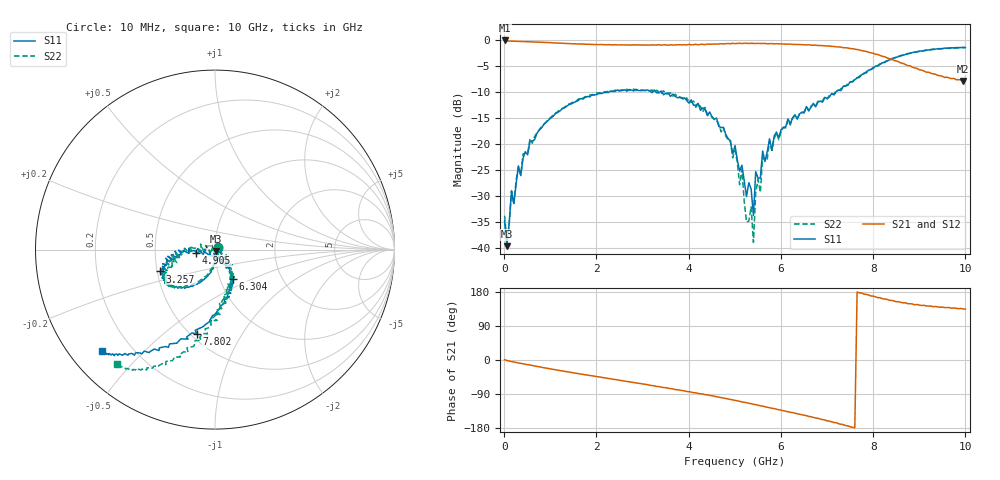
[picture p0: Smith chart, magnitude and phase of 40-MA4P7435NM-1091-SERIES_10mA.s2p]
!Agilent Technologies,E8364C,MY48140145,A.09.42.15
!Agilent E8364C: A.09.42.15
!Date: Wednesday, December 02, 2020 13:40:49
!Correction: S11(Full 2 Port(1,2))
!S21(Full 2 Port(1,2))
!S12(Full 2 Port(1,2))
!S22(Full 2 Port(1,2))
!S2P File: Measurements: S11, S21, S12, S22:
# Hz S  dB  R 50
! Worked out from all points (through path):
!   201 points, 10 MHz to 10 GHz, reference 50 ohm
!   highest |S21| = -0.11 dB at 10 MHz (marker M1); lowest = -7.9 dB at 9.95 GHz (marker M2)
!   group delay of S21, straight-line fit = 66.1 ps
!   lowest |S11| = -39.6 dB at 59.95 MHz (marker M3), VSWR 1.02, Z = 50.6 - j0.834 ohm
!   |S11| at or under -10 dB: start of sweep to 2.191 GHz; 3.293 GHz to 3.38 GHz (87.41 MHz wide, 2.62 % of centre); 3.42 GHz to 7.193 GHz (3.774 GHz wide, 71.1 % of centre)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
!   |S22| runs from -38.9 to -1.5 dB; largest |S21 - S12| = 0.021
!   S11 on the Smith chart (normalised r, x): 10 MHz: 1.03, +0.01; 3.257 GHz: 0.52, -0.14; 4.905 GHz: 0.81, -0.03; 6.304 GHz: 1.15, -0.39; 7.802 GHz: 0.54, -0.65; 10 GHz: 0.10, -0.38
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1e7  -34.80 20.2  -0.11 0.9  -0.16 -0.2  -33.77 44.9
5.995e7  -39.61 -51.9  -0.21 -1.5  -0.21 -1.6  -38.55 -59.8
1.5985e8  -29.03 -76.8  -0.24 -4.2  -0.24 -4.2  -28.99 -74.5
5.5945e8  -19.49 -97.6  -0.38 -13.6  -0.38 -13.6  -19.00 -97.4
1.7083e9  -11.37 -129.0  -0.80 -38.0  -0.78 -37.8  -11.18 -132.1
3.25675e9  -9.62 -158.4  -0.99 -68.2  -0.96 -68.9  -10.12 -150.0
3.35665e9  -10.17 -159.8  -0.94 -70.3  -0.96 -70.7  -9.99 -150.4
4.9051e9  -19.52 -169.8  -0.74 -104.3  -0.72 -103.8  -19.30 173.2
5.005e9  -20.30 177.0  -0.72 -106.6  -0.67 -106.6  -21.23 158.7
5.15485e9  -24.06 -171.5  -0.70 -110.6  -0.66 -110.5  -24.86 156.6
5.25475e9  -30.08 -167.5  -0.65 -112.8  -0.62 -113.0  -34.99 133.7
5.35465e9  -28.63 -88.2  -0.65 -115.2  -0.66 -115.3  -32.07 -59.1
5.4046e9  -33.69 -105.3  -0.67 -116.8  -0.65 -117.0  -38.88 29.5
5.45455e9  -25.30 -80.0  -0.69 -117.9  -0.69 -117.8  -29.38 -57.6
5.55445e9  -26.53 -67.0  -0.70 -120.8  -0.68 -120.8  -29.27 -28.6
5.6044e9  -21.33 -59.9  -0.70 -121.6  -0.72 -121.6  -22.53 -47.6
6.3037e9  -14.36 -58.1  -0.87 -140.3  -0.86 -140.3  -14.62 -54.6
6.7033e9  -12.17 -68.7  -1.02 -151.4  -1.01 -151.5  -12.41 -67.1
7.8022e9  -6.38 -102.3  -2.15 173.9  -2.09 174.5  -6.51 -98.0
8.35165e9  -3.84 -119.0  -3.60 157.5  -3.52 158.6  -3.90 -110.5
9.95005e9  -1.43 -137.5  -7.91 134.7  -7.80 135.6  -1.51 -130.3
1e10  -1.45 -137.9  -7.85 134.4  -7.84 134.3  -1.51 -130.7
